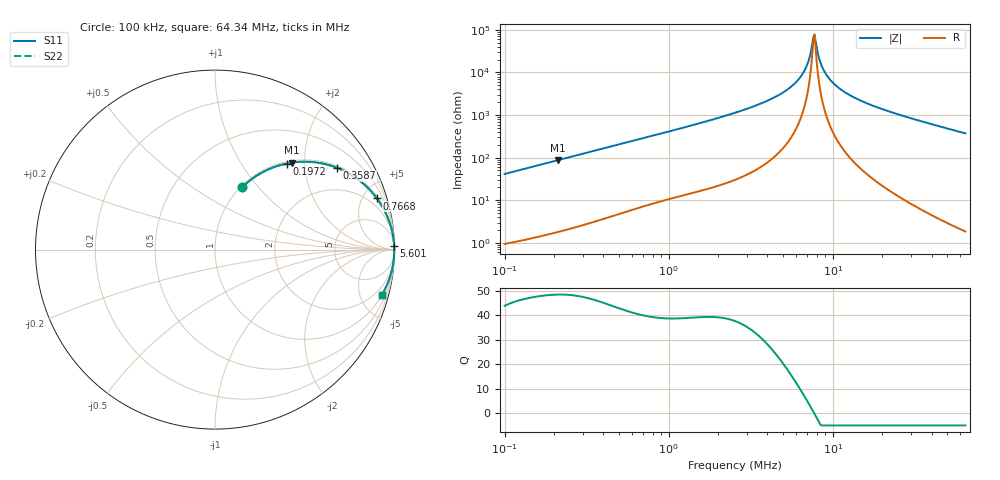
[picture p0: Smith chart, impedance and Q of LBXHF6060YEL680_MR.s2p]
! LBXHF6060YEL680_MR  S-PARAMETER MODEL  ( General Type )
! Model Generated by TAIYO YUDEN Corporation (http://www.ty-top.com)
! Version 1.0
! TAIYO YUDEN Control No. 20211118
! Copyright(c) 2021 TAIYO YUDEN CO.,LTD. All Rights Reserved.
! Product Description (link to TY-COMPAS)
! https://ds.yuden.co.jp/TYCOMPAS/or/detail?pn=LBXHF6060YEL680MMR&u=M
! Products Name : Inductors
! Characteristics :
!  Inductance : 68 uH , SRF(min) : 5.5 MHz , DC Resistance(max) : 0.385 Ohm
!  Rated Current : Saturation :1200 mA , Temp Rise : 650 mA
!  Case Size : 6.0 x 6.0 / 0.236 x 0.236 [mm/inch] , Thickness : 4.5 / 0.177 [mm/inch]
!  (Conditions: Temperature = 25 degC , DC Bias Current/Voltage = 0A / 0V)
! External Node Assignments :
!  1  o---GGG---o  2
! GND o---------o GND
! Frequency Range : 0.1MHz  -  64.339822MHz  [ 402 STEP ]
# MHz S RI R 50
! Freq[MHz].  S11 Real  S11 Imag  S21 Real  S21 Imag  S12 Real  S12 Imag  S22 Real  S22 Imag
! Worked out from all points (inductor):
!   401 points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, 100 kHz to 64.34 MHz, reference 50 ohm
!   read as one part in series: L = 65.8 uH near 103.3 kHz
!   highest Q = 48.4 at 210.4 kHz (marker M1), where L = 65.6 uH
!   self-resonance near 7.615 MHz
!   S11 on the Smith chart (normalised r, x): 100 kHz: 1.02, +0.83; 197.2 kHz: 1.03, +1.63; 358.7 kHz: 1.06, +2.94; 766.8 kHz: 1.16, +6.27; 5.601 MHz: 7, +94; 64.34 MHz: 1.04, -7.43
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0.1  0.1521 0.3479  0.8479 -0.3479  0.8479 -0.3479  0.1521 0.3479
0.197192  0.4001 0.4797  0.5999 -0.4797  0.5999 -0.4797  0.4001 0.4797
0.210366  0.4306 0.4849  0.5694 -0.4849  0.5694 -0.4849  0.4306 0.4849
0.295407  0.5941 0.4807  0.4059 -0.4807  0.4059 -0.4807  0.5941 0.4807
0.358653  0.6808 0.4555  0.3192 -0.4555  0.3192 -0.4555  0.6808 0.4555
0.766781  0.9019 0.2851  0.0981 -0.2851  0.0981 -0.2851  0.9019 0.2851
0.872651  0.9217 0.2561  0.0783 -0.2561  0.0783 -0.2561  0.9217 0.2561
2.53653  0.99 0.0872  0.01 -0.0872  0.01 -0.0872  0.99 0.0872
4.119798  0.9965 0.0434  0.00349 -0.0434  0.00349 -0.0434  0.9965 0.0434
5.601169  0.9982 0.0211  0.00183 -0.0211  0.00183 -0.0211  0.9982 0.0211
6.272304  0.9985 0.0135  0.00151 -0.0135  0.00151 -0.0135  0.9985 0.0135
6.800379  0.9986 0.00818  0.00136 -0.00818  0.00136 -0.00818  0.9986 0.00818
7.138331  0.9987 0.005  0.0013 -0.005  0.0013 -0.005  0.9987 0.005
7.493079  0.9987 0.00183  0.00126 -0.00183  0.00126 -0.00183  0.9987 0.00183
7.615203  0.9987 0.000777  0.00125 -0.000777  0.00125 -0.000777  0.9987 0.000777
7.865456  0.9988 -0.00133  0.00125 0.00133  0.00125 0.00133  0.9988 -0.00133
8.390903  0.9987 -0.00556  0.00126 0.00556  0.00126 0.00556  0.9987 -0.00556
8.807898  0.9987 -0.00874  0.00129 0.00874  0.00129 0.00874  0.9987 -0.00874
10.52217  0.9984 -0.0206  0.00161 0.0206  0.00161 0.0206  0.9984 -0.0206
14.07625  0.9971 -0.0417  0.0029 0.0417  0.0029 0.0417  0.9971 -0.0417
22.13506  0.9921 -0.0818  0.00789 0.0818  0.00789 0.0818  0.9921 -0.0818
64.33982  0.9314 -0.2504  0.0686 0.2504  0.0686 0.2504  0.9314 -0.2504
